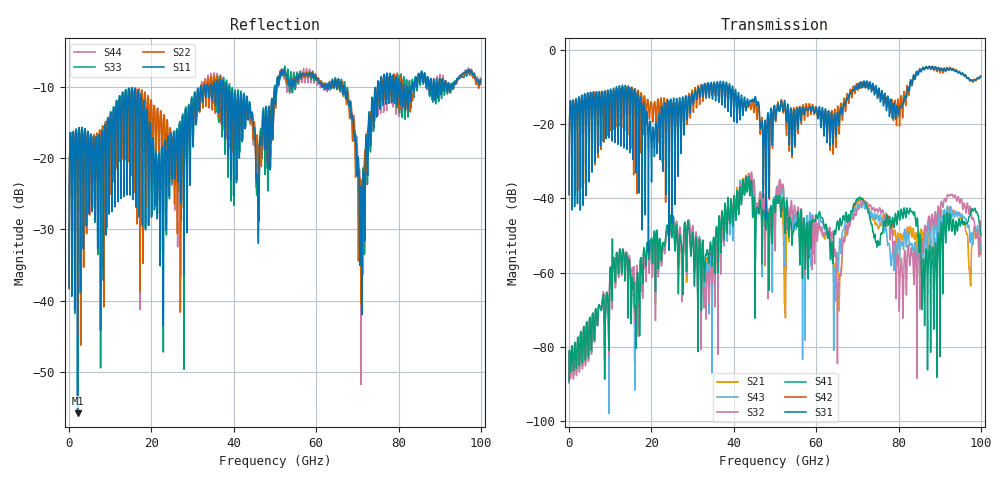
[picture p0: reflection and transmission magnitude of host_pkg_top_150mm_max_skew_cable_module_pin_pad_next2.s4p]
# Hz S RI R 50
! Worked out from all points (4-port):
!   10000 points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, 10 MHz to 100 GHz, reference 50 ohm
!   strongest paths, dB at 10 MHz, 25.01 GHz, 50.01 GHz, 75.01 GHz, 100 GHz:
!     S31: -38.9, -32.6, -16.8, -11.7, -7.0
!     S42: -39.1, -23.6, -16.0, -11.7, -6.9
!     S41: -89.3, -49.9, -42.4, -51.8, -49.9
!     S32: -89.9, -48.8, -48.4, -43.6, -46.1
!     S43: -89.6, -49.3, -42.1, -44.8, -54.2
!     S21: -89.6, -49.2, -47.6, -47.8, -55.1
!   lowest |S11| = -55.7 dB at 2.07 GHz (marker M1), VSWR 1.00, Z = 50.1 + j0.152 ohm
!   |S11| at or under -10 dB: start of sweep to 31.93 GHz; 38.88 GHz to 49.89 GHz (11.01 GHz wide, 24.8 % of centre); 66.86 GHz to 74.94 GHz (8.072 GHz wide, 11.4 % of centre)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
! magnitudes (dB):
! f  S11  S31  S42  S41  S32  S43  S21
! 10 MHz  -38.2  -38.9  -39.1  -89.3  -89.9  -89.6  -89.6
! 2.07 GHz  -55.7  -28.3  -37.9  -77.8  -78.9  -78.4  -78.4
! 33.1 GHz  -11.0  -9.6  -11.4  -56.2  -64.6  -60.5  -57.8
! 43.27 GHz  -12.2  -13.2  -14.9  -38.0  -36.7  -37.7  -37.7
! 65.48 GHz  -9.2  -19.8  -19.2  -48.4  -62.6  -56.8  -62.5
! 71.17 GHz  -40.6  -10.0  -8.7  -39.9  -41.6  -42.5  -39.9
! 100 GHz  -9.3  -7.0  -6.9  -49.9  -46.1  -54.2  -55.1
